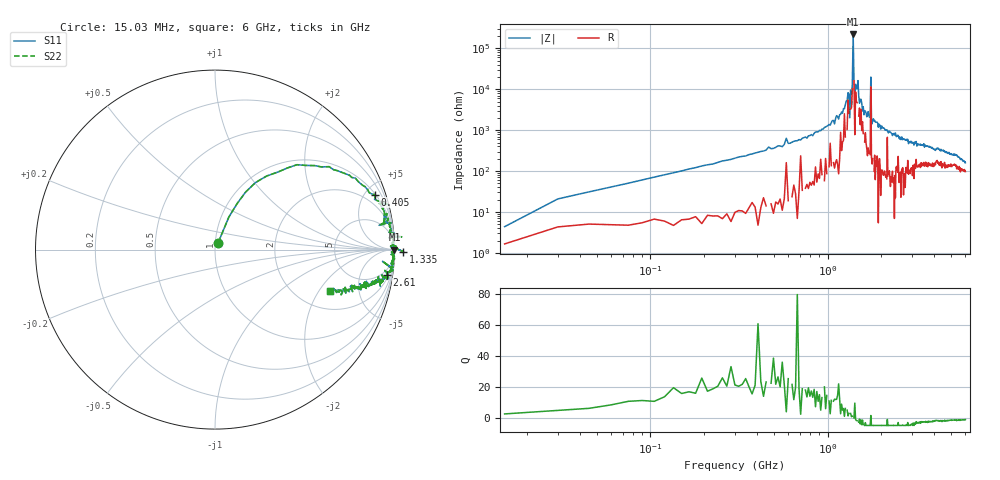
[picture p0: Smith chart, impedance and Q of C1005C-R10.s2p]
!	Network	Analyzer	HP8753E.07.74:	Oct	30	2002	Serial	No.	JP38451487
!	Hewlett-Packard
!	28	Aug	2009	9:29:53
!	Frequency	S11	S21	S12	S22
#	HZ	S	RI	R	50
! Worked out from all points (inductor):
!   400 points, 15.03 MHz to 6 GHz, reference 50 ohm
!   read as one part in series: L = 107 nH near 45.03 MHz
!   highest |Z| = 218 kohm at 1.395 GHz (marker M1)
!   self-resonance near 1.32 GHz
!   S11 on the Smith chart (normalised r, x): 15.03 MHz: 1.03, +0.08; 405 MHz: 1.10, +5.78; 1.335 GHz: -39, -9; 2.61 GHz: 3, -13; 6 GHz: 2.94, -2.55
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1.502992e7  0.0178 0.0392  0.982 -0.0392  0.982 -0.0392  0.0178 0.0392
3.002985e7  0.077 0.181  0.923 -0.181  0.923 -0.181  0.077 0.181
9.002955e7  0.288 0.41  0.712 -0.41  0.712 -0.41  0.288 0.41
4.05028e8  0.889 0.306  0.111 -0.306  0.111 -0.306  0.889 0.306
1.020025e9  0.988 0.0707  0.0117 -0.0707  0.0117 -0.0707  0.988 0.0707
1.305023e9  0.992 0.00897  0.00803 -0.00897  0.00803 -0.00897  0.992 0.00897
1.335023e9  1.05 -0.0113  -0.0508 0.0113  -0.0508 0.0113  1.05 -0.0113
1.350023e9  0.996 0.0098  0.00369 -0.0098  0.00369 -0.0098  0.996 0.0098
1.365023e9  0.98 0.0123  0.02 -0.0123  0.02 -0.0123  0.98 0.0123
1.395023e9  1 0.000183  -0.00042 -0.000183  -0.00042 -0.000183  1 0.000183
1.425023e9  0.998 0.0135  0.00162 -0.0135  0.00162 -0.0135  0.998 0.0135
1.485023e9  1 -0.00366  -0.00494 0.00366  -0.00494 0.00366  1 -0.00366
1.515022e9  0.983 -0.0137  0.0166 0.0137  0.0166 0.0137  0.983 -0.0137
1.740021e9  0.992 -0.0461  0.00772 0.0461  0.00772 0.0461  0.992 -0.0461
1.755021e9  0.997 0.00409  0.0029 -0.00409  0.0029 -0.00409  0.997 0.00409
1.785021e9  0.988 -0.0679  0.0118 0.0679  0.0118 0.0679  0.988 -0.0679
2.01002e9  0.987 -0.0774  0.0126 0.0774  0.0126 0.0774  0.987 -0.0774
2.610017e9  0.957 -0.143  0.0426 0.143  0.0426 0.143  0.957 -0.143
3.015015e9  0.937 -0.177  0.0626 0.177  0.0626 0.177  0.937 -0.177
4.00501e9  0.845 -0.206  0.155 0.206  0.155 0.206  0.845 -0.206
5.010005e9  0.776 -0.21  0.224 0.21  0.224 0.21  0.776 -0.21
6e9  0.642 -0.231  0.358 0.231  0.358 0.231  0.642 -0.231
